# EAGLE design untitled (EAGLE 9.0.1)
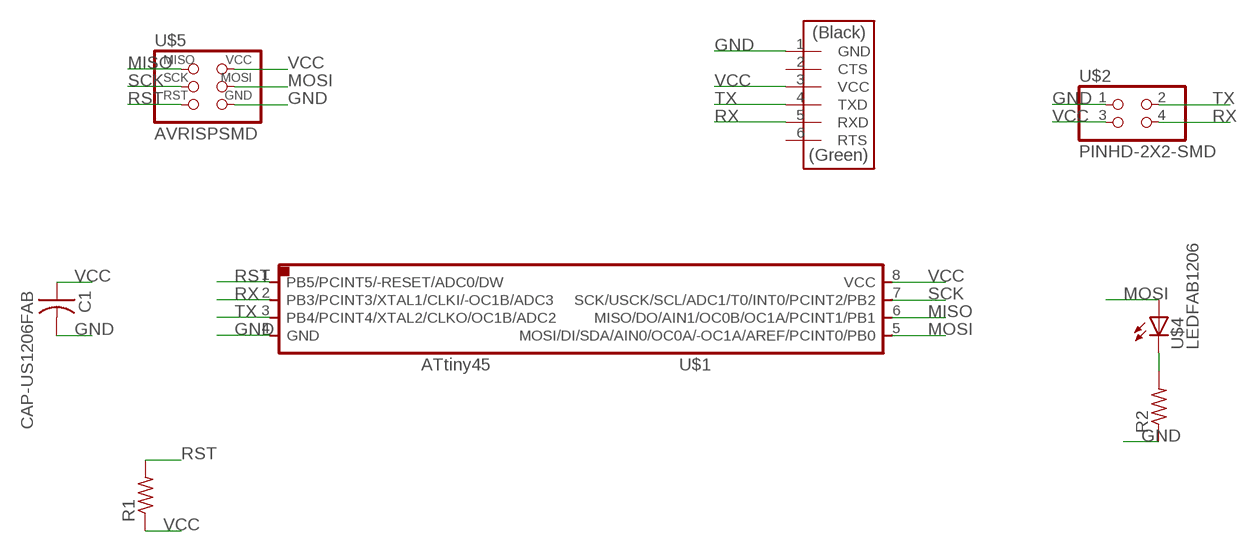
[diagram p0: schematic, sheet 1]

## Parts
C1  CAP-US1206FAB  [C1206FAB]
R1  RES-US1206FAB  [R1206FAB]
R2  RES-US1206FAB  [R1206FAB]
U$1  ATTINY45SI  [SOIC8]
U$2  PINHD-2X2-SMD  [2X02SMD]
U$3  FTDI-SMD-HEADER  [1X06SMD]
U$4  LEDFAB1206  [LED1206FAB]
U$5  AVRISPSMD  [2X03SMD]

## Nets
GND: C1.2 R2.1 U$1.4(GND) U$2.1 U$3.1(GND) U$5.6(GND)
MISO: U$1.6(MISO/DO/AIN1/OC0B/OC1A/PCINT1/PB1) U$5.1(MISO)
MOSI: U$1.5(MOSI/DI/SDA/AIN0/OC0A/-OC1A/AREF/PCINT0/PB0) U$4.1(A) U$5.4(MOSI)
N$5: R2.2 U$4.2(C)
RST: R1.2 U$1.1(PB5/PCINT5/-RESET/ADC0/DW) U$5.5(RST)
RX: U$1.2(PB3/PCINT3/XTAL1/CLKI/-OC1B/ADC3) U$2.4 U$3.5(RXD)
SCK: U$1.7(SCK/USCK/SCL/ADC1/T0/INT0/PCINT2/PB2) U$5.3(SCK)
TX: U$1.3(PB4/PCINT4/XTAL2/CLKO/OC1B/ADC2) U$2.2 U$3.4(TXD)
VCC: C1.1 R1.1 U$1.8(VCC) U$2.3 U$3.3(VCC) U$5.2(VCC)
Unconnected: U$3.2(CTS) U$3.6(RTS)

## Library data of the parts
C1 = fab:CAP-US
R1 R2 = fab:RES-US: Resistor (US Symbol)
U$1 = fab:ATTINY45
U$2 = fab:PINHD-2X2-SMD
U$3 = fab:FTDI-SMD-HEADER
U$4 = fab:LED: LED
U$5 = fab:AVRISP

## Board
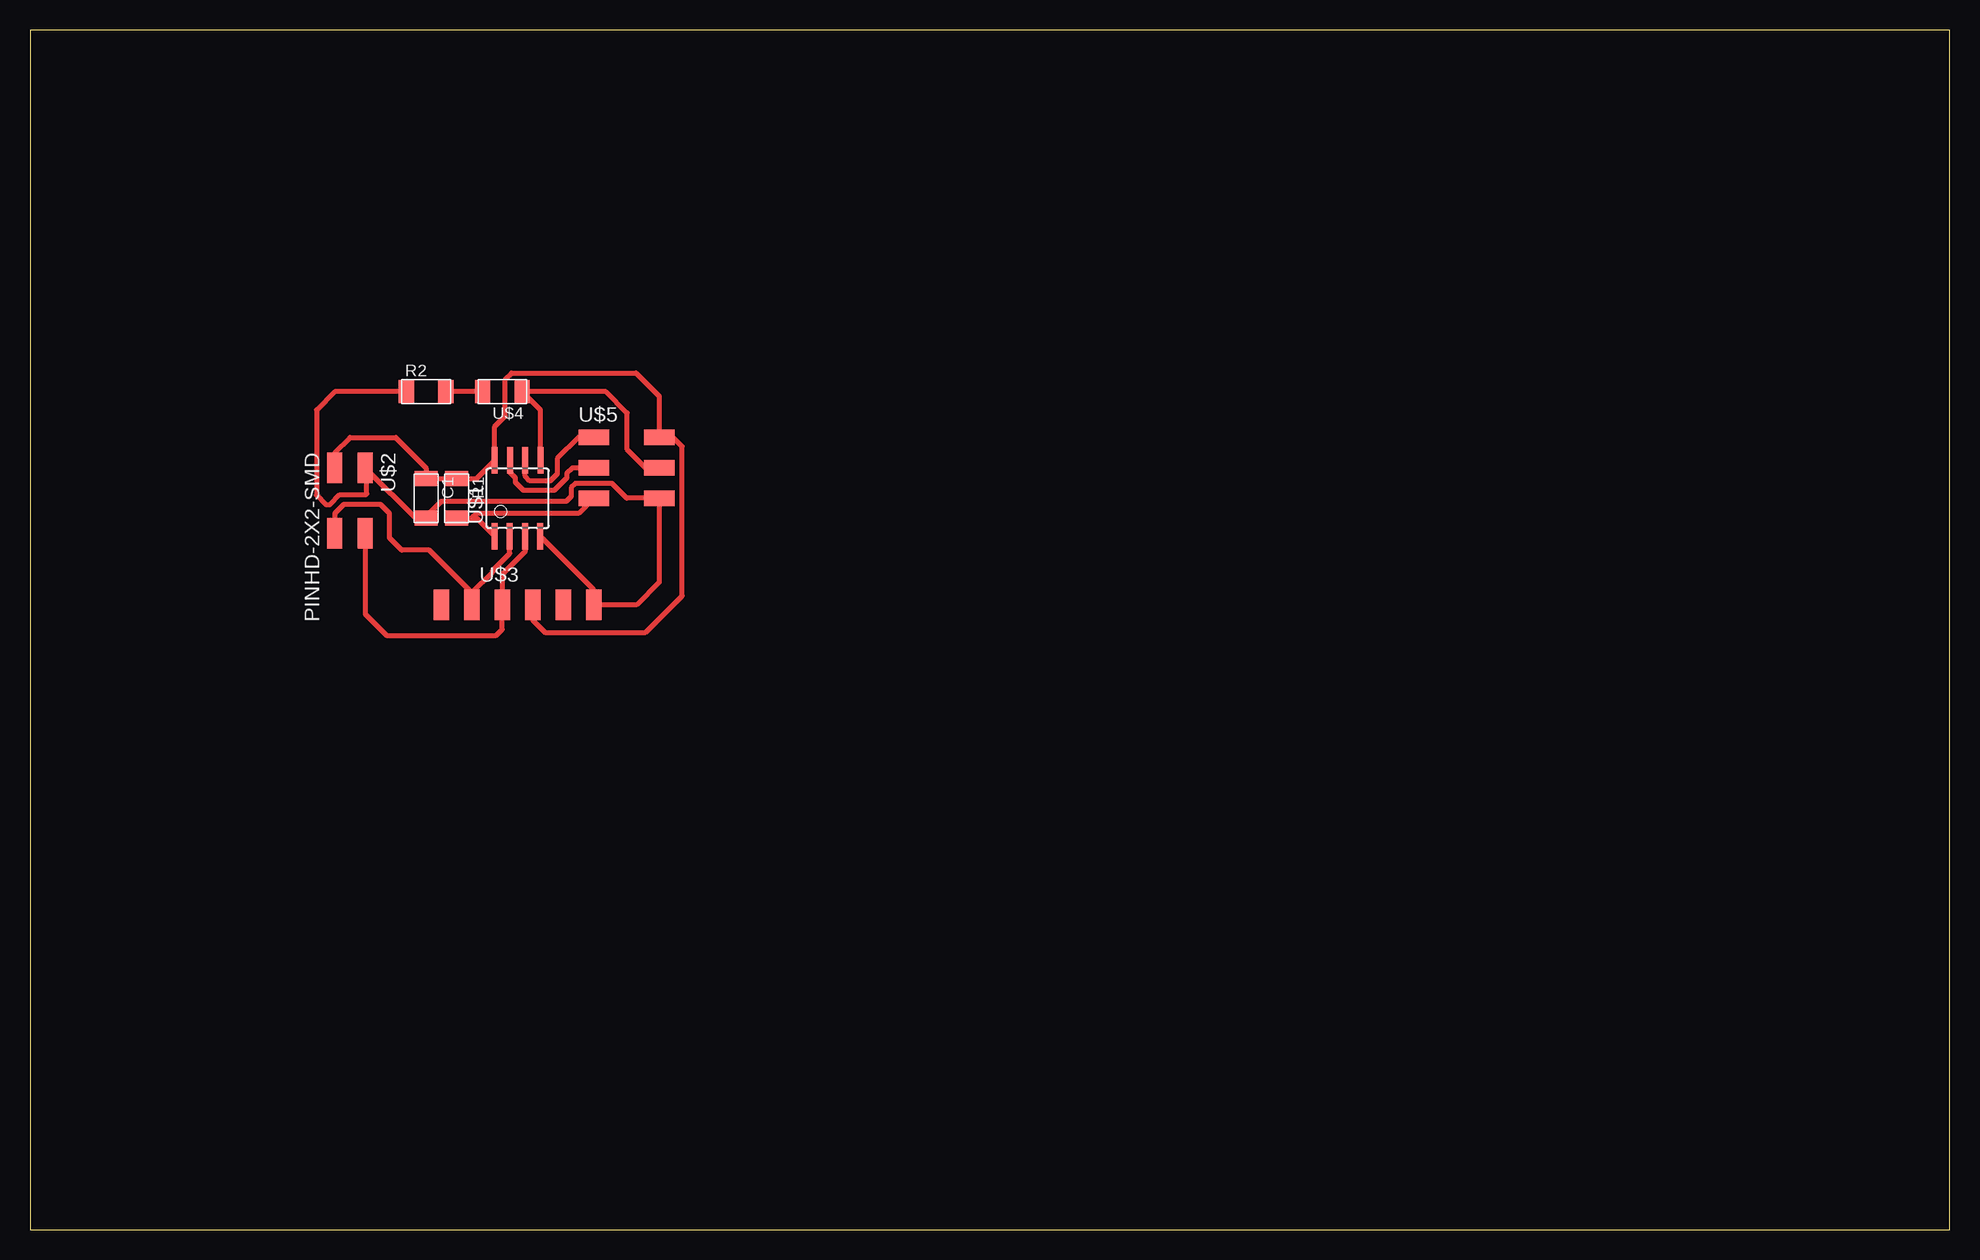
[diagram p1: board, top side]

Size 160 x 100 mm. Coordinates in mm from the lower left corner, seen from the top.
Outline: 0,0 160,0 160,100 0,100 0,0
Copper layers (1*16): Top 0.035mm / dielectric 1.5mm / Bottom 0.035mm
Design rules "default *": minimum track width 0.4mm, minimum drill 0.35mm, track to track 0.4mm, track to pad 0.4mm, pad to pad 0.4mm, via to via 0.4mm, smd to smd 6mil, copper to edge 40mil, drill to drill 6mil, minimum pad ring 10mil, minimum via ring 8mil, stop-mask expansion 4mil, vias tented up to drill 0mil, thermal gap 10mil

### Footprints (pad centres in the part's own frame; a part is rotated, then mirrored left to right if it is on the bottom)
C1206FAB = smd 1.27 x 1.905: 1 -1.651,0; 2 1.651,0
R1206FAB = smd 1.27 x 1.905: 1 -1.651,0; 2 1.651,0
SOIC8 = smd 0.5 x 2.2: 1 -1.905,-3.154; 2 -0.645,-3.154; 3 0.625,-3.154; 4 1.895,-3.154; 5 1.905,3.154; 6 0.635,3.154; 7 -0.635,3.154; 8 -1.905,3.154
2X02SMD = smd 2.54 x 1.27: 1 -2.54,1.27; 2 2.92,1.27; 3 -2.54,-1.27; 4 2.92,-1.27
1X06SMD = smd 2.54 x 1.27: 1 0,6.35; 2 0,3.81; 3 0,1.27; 4 0,-1.27; 5 0,-3.81; 6 0,-6.35
LED1206FAB = smd 1.27 x 1.905: 1 -1.651,0; 2 1.651,0
2X03SMD = smd 2.54 x 1.27: 1 -2.54,2.54; 2 2.92,2.54; 3 -2.54,0; 4 2.92,0; 5 -2.54,-2.54; 6 2.92,-2.54

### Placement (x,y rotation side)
C1  33.02,60.96 270 top
R1  35.56,60.96 270 top
R2  33.02,69.85 0 top
U$1  40.64,60.96 0 top
U$2  26.67,60.96 270 top
U$3  40.64,52.07 270 top
U$4  39.37,69.85 180 top
U$5  49.53,63.5 0 top

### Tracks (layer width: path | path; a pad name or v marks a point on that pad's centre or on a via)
GND
  Top 0.4: U$2.1 28.07,63.37 | 28.07,63.37 32.13,59.31 C1.2 33.02,59.44 34.29,60.71 44.7,60.71 45.12,61.12 45.12,61.84 45.47,62.2 48.51,62.2 49.74,60.96 U$5.6 52.45,53.97 50.55,52.07 U$3.1 46.99,53.34 42.53,57.8 U$1.4 | R2.1 25.4,69.85 23.88,68.33 23.88,61.21 24.64,60.45 25.03,60.45 25.83,61.25 27.98,61.25 28.07,61.34 28.07,63.37
MISO
  Top 0.4: U$5.1 45.72,66.04 43.94,64.26 43.94,62.99 43.36,62.41 41.66,62.41 41.27,62.8 U$1.6
MOSI
  Top 0.4: U$1.5 42.55,68.33 U$4.1 48.01,69.85 49.78,68.07 49.78,65.02 51.31,63.5 U$5.4
N$5
  Top 0.4: U$4.2 R2.2
RST
  Top 0.4: R1.2 36.83,59.31 | 36.83,59.31 37.23,59.31 U$1.1 | U$5.5 45.72,59.69 37.21,59.69 36.83,59.31
RX
  Top 0.4: 36.83,53.09 33.27,56.64 30.99,56.64 29.97,57.66 29.97,59.69 29.21,60.45 26.16,60.45 25.4,59.69 U$2.4 | U$3.5 36.83,53.09 | 36.83,53.09 38.57,54.83 38.57,54.94 39.99,56.37 U$1.2
SCK
  Top 0.4: U$5.3 45.21,63.5 44.74,63.03 44.74,62.66 43.7,61.61 41.14,61.61 40.48,62.28 40.48,62.65 40.01,63.12 U$1.7
TX
  Top 0.4: U$2.2 27.94,51.31 29.72,49.53 38.86,49.53 39.37,50.04 U$3.4 39.37,54.61 41.27,56.51 U$1.3
VCC
  Top 0.4: U$2.3 25.4,64.77 26.67,66.04 30.48,66.04 33.02,63.5 C1.1 R1.1 37.23,62.61 U$1.8 38.73,66.93 39.62,67.82 39.62,70.89 40.14,71.4 50.52,71.4 52.45,69.47 U$5.2 53.59,66.04 54.36,65.28 54.36,52.83 51.31,49.78 42.93,49.78 41.91,50.8 U$3.3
